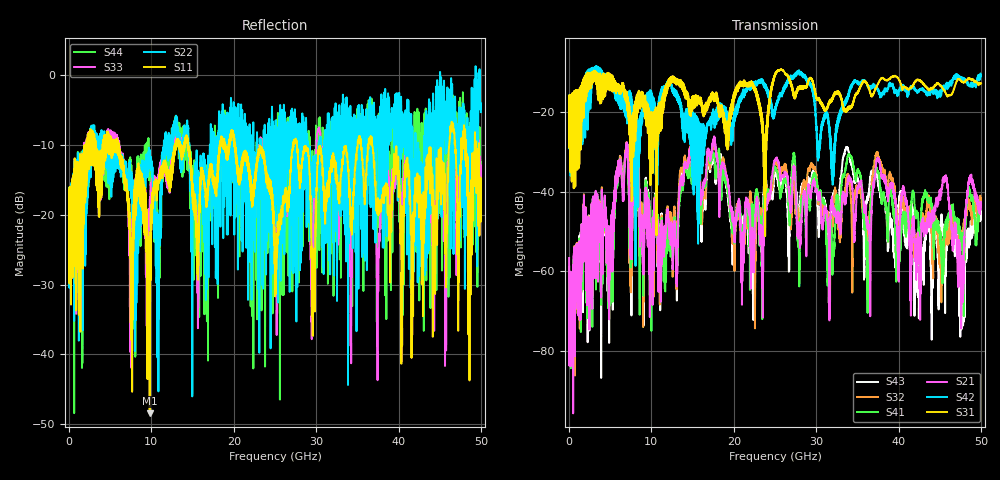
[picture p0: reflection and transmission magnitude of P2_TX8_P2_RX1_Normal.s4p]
!Keysight Technologies,N5225B,MY57041031,A.13.20.10
!Date: Friday, May 31, 2019 11:28:04
!Correction: S11(Full 4 Port(1,2,3,4))
!S12(Full 4 Port(1,2,3,4))
!S13(Full 4 Port(1,2,3,4))
!S14(Full 4 Port(1,2,3,4))
!S21(Full 4 Port(1,2,3,4))
!S22(Full 4 Port(1,2,3,4))
!S23(Full 4 Port(1,2,3,4))
!S24(Full 4 Port(1,2,3,4))
!S31(Full 4 Port(1,2,3,4))
!S32(Full 4 Port(1,2,3,4))
!S33(Full 4 Port(1,2,3,4))
!S34(Full 4 Port(1,2,3,4))
!S41(Full 4 Port(1,2,3,4))
!S42(Full 4 Port(1,2,3,4))
!S43(Full 4 Port(1,2,3,4))
!S44(Full 4 Port(1,2,3,4))
!S4P File: Measurements: <S11,S12,S13,S14>,
!<S21,S22,S23,S24>,
!<S31,S32,S33,S34>,
!<S41,S42,S43,S44>:
# Hz S  dB  R 50.0
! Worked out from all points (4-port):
!   5000 points, 10 MHz to 50 GHz, reference 50 ohm
!   strongest paths, dB at 10 MHz, 12.51 GHz, 25.01 GHz, 37.51 GHz, 50 GHz:
!     S31: -19.3, -11.5, -10.3, -12.8, -12.8
!     S42: -19.4, -14.3, -20.0, -14.4, -10.9
!     S21: -56.7, -50.0, -32.1, -31.9, -43.2
!     S41: -63.2, -50.2, -34.0, -34.9, -42.9
!     S32: -77.6, -49.7, -32.4, -30.6, -42.7
!     S43: -58.9, -49.7, -35.1, -37.9, -45.8
!   lowest |S11| = -48.4 dB at 9.79 GHz (marker M1), VSWR 1.01, Z = 49.9 - j0.358 ohm
!   |S11| at or under -10 dB: 20.17 GHz to 27.18 GHz (7.009 GHz wide, 29.6 % of centre); 27.67 GHz to 35.04 GHz (7.368 GHz wide, 23.5 % of centre); 36.79 GHz to 46.15 GHz (9.363 GHz wide, 22.6 % of centre)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
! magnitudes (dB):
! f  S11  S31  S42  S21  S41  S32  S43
! 10 MHz  -19.7  -19.3  -19.4  -56.7  -63.2  -77.6  -58.9
! 6.94 GHz  -16.5  -16.2  -21.3  -28.8  -29.2  -28.4  -29.1
! 9.79 GHz  -48.4  -26.0  -18.8  -48.2  -46.3  -47.0  -45.3
! 17.57 GHz  -15.8  -17.2  -22.8  -26.5  -30.4  -27.4  -32.2
! 21.05 GHz  -11.7  -13.3  -15.1  -60.8  -51.0  -54.9  -48.2
! 25.14 GHz  -25.8  -10.1  -17.9  -31.6  -34.3  -32.8  -35.9
! 50 GHz  -14.9  -12.8  -10.9  -43.2  -42.9  -42.7  -45.8
